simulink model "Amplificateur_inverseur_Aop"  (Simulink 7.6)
settings: Solver=ode23t  StartTime=0.0  StopTime=0.04  RelTol=1e-3
InitFcn:
  | clc
  | clear all
  | close all
  | delete *.mat
libraries: powerlib x18

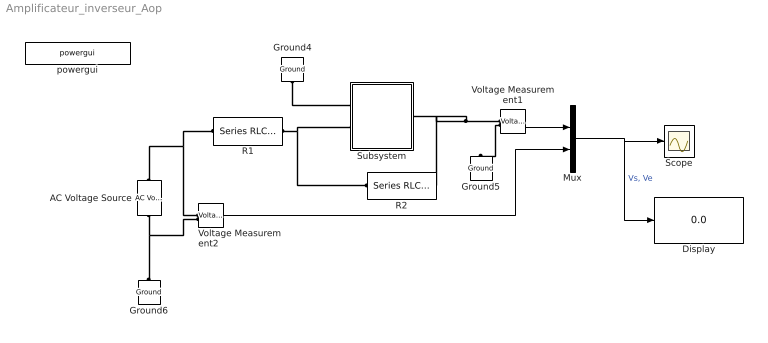
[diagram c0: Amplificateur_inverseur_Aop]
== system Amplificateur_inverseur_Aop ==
  AC Voltage Source : powerlib/Electrical Sources/AC Voltage Source  DialogController=POWERSYS.PowerSysDialog  SystemSampleTime=-1  Amplitude=0.1  Phase=0  Frequency=60  SampleTime=0  Measurements=None
  Display : Display
  Ground4 : powerlib/Elements/Ground  DialogController=POWERSYS.PowerSysDialog  PhysicalDomain=powersysdomain  SubClassName=unknown  LeftPortType=p1  RightPortType=p1  LConnTagsString=a
  Ground5 : powerlib/Elements/Ground  DialogController=POWERSYS.PowerSysDialog  PhysicalDomain=powersysdomain  SubClassName=unknown  LeftPortType=p1  RightPortType=p1  LConnTagsString=a
  Ground6 : powerlib/Elements/Ground  DialogController=POWERSYS.PowerSysDialog  PhysicalDomain=powersysdomain  SubClassName=unknown  LeftPortType=p1  RightPortType=p1  LConnTagsString=a
  Mux : Mux  Inputs=2
  R1 : powerlib/Elements/Series RLC Branch  DialogController=POWERSYS.PowerSysDialog  PhysicalDomain=powersysdomain  SubClassName=unknown  LeftPortType=p1  RightPortType=p1  LConnTagsString=__new0  RConnTagsString=__new0  BranchType=R  Resistance=10e3  Inductance=10e-3  SetiL0=off  InitialCurrent=0  Capacitance=0  Setx0=off  InitialVoltage=0  Measurements=None
  R2 : powerlib/Elements/Series RLC Branch  DialogController=POWERSYS.PowerSysDialog  PhysicalDomain=powersysdomain  SubClassName=unknown  LeftPortType=p1  RightPortType=p1  LConnTagsString=__new0  RConnTagsString=__new0  BranchType=R  Resistance=100e3  Inductance=10e-3  SetiL0=off  InitialCurrent=0  Capacitance=0  Setx0=off  InitialVoltage=0  Measurements=None
  Scope : Scope
  Subsystem : Subsystem
  Voltage Measurement1 : powerlib/Measurements/Voltage Measurement  DialogController=POWERSYS.PowerSysDialog  SystemSampleTime=-1  PhasorSimulation=off  OutputType=Complex  PSBequivalent=0
  Voltage Measurement2 : powerlib/Measurements/Voltage Measurement  DialogController=POWERSYS.PowerSysDialog  SystemSampleTime=-1  PhasorSimulation=off  OutputType=Complex  PSBequivalent=0
  powergui : powerlib/powergui  Priority=1  SystemSampleTime=-1  SimulationMode=Continuous  SampleTime=50e-6  frequency=60  SPID=off  DisableSnubberDevices=off  DisableRonSwitches=off  DisableVfSwitches=off  SwTol=0  Interpol=off  frequencyindice=0  echomessages=off  HookPort=off  DisplayEquations=off  FunctionMessages=off  EnableUseOfTLC=off  x0status=blocks  RestoreLinks=warning  ResistiveCurrentMeasurement=off  Ylog=off  Xlog=on  ShowGrid=off  save=off  variable=ZData  ZoomFFT=off  StartTime=0.0  cycles=1  DisplayStyle=1  fundamental=60  FreqAxis=off  MaxFrequency=1000  frequencyindicesteady=1  display=off  methode=off
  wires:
  Voltage Measurement1/1 -> Mux/1
  Mux/1 -> Scope/1, Display/1  "Vs, Ve"
  Voltage Measurement2/1 -> Mux/2
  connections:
  Ground4/LConn1 -- Subsystem/LConn1
  Voltage Measurement1/LConn1 -- Subsystem/RConn1 -- R2/RConn1
  R1/RConn1 -- Subsystem/LConn2 -- R2/LConn1
  Voltage Measurement1/LConn2 -- Ground5/LConn1
  AC Voltage Source/RConn1 -- R1/LConn1 -- Voltage Measurement2/LConn1
  AC Voltage Source/LConn1 -- Ground6/LConn1 -- Voltage Measurement2/LConn2

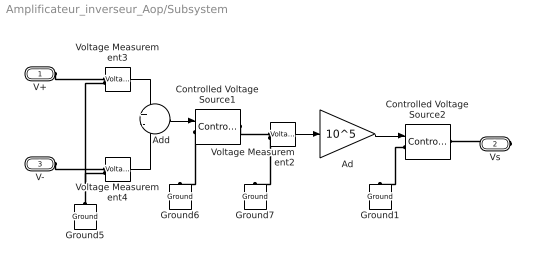
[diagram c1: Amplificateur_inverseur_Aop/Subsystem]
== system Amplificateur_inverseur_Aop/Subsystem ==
  Ad : Gain  Gain=10^5
  Add : Sum  Inputs=+-
  Controlled Voltage Source1 : powerlib/Electrical Sources/Controlled Voltage Source  DialogController=POWERSYS.PowerSysDialog  SystemSampleTime=-1  Initialize=on  Source_Type=AC  Amplitude=0  Phase=0  Frequency=0  Measurements=None
  Controlled Voltage Source2 : powerlib/Electrical Sources/Controlled Voltage Source  DialogController=POWERSYS.PowerSysDialog  SystemSampleTime=-1  Initialize=on  Source_Type=AC  Amplitude=0  Phase=0  Frequency=0  Measurements=None
  Ground{1,5..7} (4 alike) : powerlib/Elements/Ground  DialogController=POWERSYS.PowerSysDialog  PhysicalDomain=powersysdomain  SubClassName=unknown  LeftPortType=p1  RightPortType=p1  LConnTagsString=a
  Voltage Measurement2 : powerlib/Measurements/Voltage Measurement  DialogController=POWERSYS.PowerSysDialog  SystemSampleTime=-1  PhasorSimulation=off  OutputType=Complex  PSBequivalent=0
  Voltage Measurement3 : powerlib/Measurements/Voltage Measurement  DialogController=POWERSYS.PowerSysDialog  SystemSampleTime=-1  PhasorSimulation=off  OutputType=Complex  PSBequivalent=0
  Voltage Measurement4 : powerlib/Measurements/Voltage Measurement  DialogController=POWERSYS.PowerSysDialog  SystemSampleTime=-1  PhasorSimulation=off  OutputType=Complex  PSBequivalent=0
  V+ : PMIOPort  Port=1  Side=Left
  Vs : PMIOPort  Port=2  Side=Right
  V- : PMIOPort  Port=3  Side=Left
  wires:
  Ad/1 -> Controlled Voltage Source2/1
  Voltage Measurement3/1 -> Add/1
  Voltage Measurement4/1 -> Add/2
  Voltage Measurement2/1 -> Ad/1
  Add/1 -> Controlled Voltage Source1/1
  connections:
  V-/RConn1 -- Voltage Measurement4/LConn1
  Vs/RConn1 -- Controlled Voltage Source2/RConn1
  V+/RConn1 -- Voltage Measurement3/LConn1
  Voltage Measurement2/LConn2 -- Ground7/LConn1
  Ground5/LConn1 -- Voltage Measurement4/LConn2 -- Voltage Measurement3/LConn2
  Controlled Voltage Source2/LConn1 -- Ground1/LConn1
  Controlled Voltage Source1/RConn1 -- Voltage Measurement2/LConn1
  Controlled Voltage Source1/LConn1 -- Ground6/LConn1
